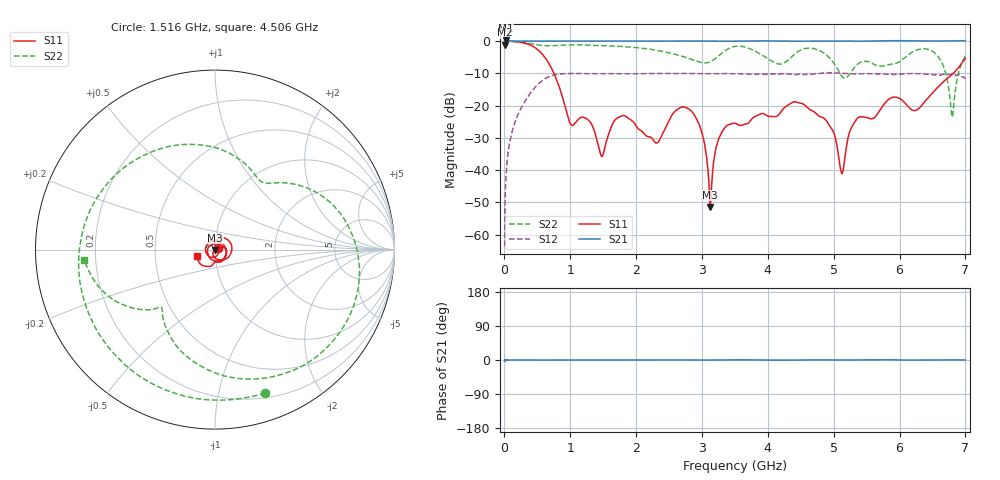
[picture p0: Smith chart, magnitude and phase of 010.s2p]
!Keysight Technologies,N5232A,MY52221221,A.10.65.11
!Date: Wednesday, October 16, 2024 11:57:18
!Correction: S11(Full 2 Port(1,4))
!S41(Full 2 Port(1,4))
!S14(Full 2 Port(1,4))
!S44(Full 2 Port(1,4))
!S2P File: Measurements: S11, S41, S14, S44:
# Hz S  RI  R 50
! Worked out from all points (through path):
!   4000 points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, 2.05 MHz to 7 GHz, reference 50 ohm
!   highest |S21| = 0.20 dB at 17.8 MHz (marker M1); lowest = -1.2 dB at 2.05 MHz (marker M2)
!   lowest |S11| = -51.4 dB at 3.126 GHz (marker M3), VSWR 1.01, Z = 50 - j0.266 ohm
!   |S11| at or under -10 dB: 750.9 MHz to 6.816 GHz (6.065 GHz wide, 160 % of centre)
!   |S22| runs from -23.6 to 0.0 dB; largest |S21 - S12| = 1.3
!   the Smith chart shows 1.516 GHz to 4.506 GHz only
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2049925  -0.9685 0.1509  0.8745 -0.045  0.000142 0.000647  -0.9768 0.098
1.779925e7  -0.9865 0.1505  1.023 0.00832  0.000837 0.00611  -0.9981 0.0599
1.840421e8  -0.0076 0.9766  0.9978 0.00158  0.0618 0.0187  -0.8067 0.5524
3.415354e8  0.8923 0.1671  0.9992 0.00136  0.0874 -0.0978  -0.4304 0.8289
4.867792e8  0.2802 -0.7083  0.9995 -0.000885  -0.0805 -0.1876  -0.0507 0.8791
6.320229e8  -0.4582 -0.2592  0.9971 0.00123  -0.2679 0.00989  0.2691 0.8047
1.16925e9  0.0306 0.0583  0.999 0.00314  0.1637 -0.2661  0.8451 -0.2187
1.478987e9  0.0163 0.00164  0.9995 0.00162  -0.3121 0.0121  0.3604 -0.7681
1.690728e9  0.0616 -0.00284  0.998 0.00254  -0.0252 0.3103  -0.1307 -0.8249
2.3347e9  0.00076 0.0271  1.001 0.00417  -0.286 -0.1301  -0.6406 0.3139
2.828179e9  0.071 -0.0453  1.003 0.00111  0.3053 0.0725  0.1214 0.5122
3.125666e9  0.000338 -0.00266  0.9989 -0.00139  -0.0598 -0.306  0.3035 0.37
3.5019e9  -0.0524 0.00909  0.9974 0.00763  -0.1253 0.2855  0.7928 -0.2387
3.795887e9  0.0647 -0.0187  1.008 0.0044  0.3088 0.00437  0.0622 -0.7067
4.261367e9  -0.022 -0.0923  0.9998 -0.00672  -0.3075 -0.0115  -0.3328 -0.329
4.66735e9  -0.0822 0.0171  0.9968 0.00437  0.2706 0.1439  -0.6181 0.4612
5.12583e9  0.00765 -0.00442  1.003 0.00133  -0.281 -0.1503  0.1522 0.2407
5.446067e9  -0.0606 0.0281  0.9955 0.00553  0.0296 0.3112  0.3855 0.2891
5.83455e9  -0.0816 0.0944  1.012 0.0117  0.1195 -0.2815  0.4073 -0.1416
6.499521e9  0.0104 0.1561  1.004 -3.17e-05  0.2685 0.1383  -0.6385 -0.2751
6.800509e9  0.2872 -0.1022  1.008 0.00469  -0.0404 -0.31  -0.0662 -0.0022
7e9  -0.4453 -0.3086  1.014 0.00088  -0.2541 0.055  -0.5836 -0.0496
